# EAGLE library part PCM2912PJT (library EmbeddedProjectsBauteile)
TEXAS INSTRUMENTS PCM2912PJT - AUDIO CODEC, USB INTERFACE 32TQFP
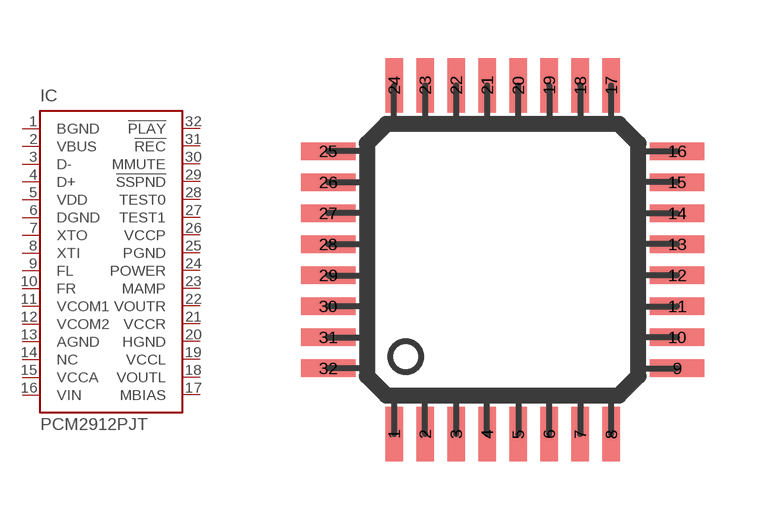
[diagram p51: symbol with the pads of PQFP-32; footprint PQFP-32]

Designator prefix IC

## PCM2912PJT  [PQFP-32]
1  BGND  pwr
2  VBUS  pwr
3  D-
4  D+
5  VDD  pwr
6  DGND  pwr
7  XTO  out
8  XTI  in
9  FL  in
10  FR  in
11  VCOM1  pwr
12  VCOM2  pwr
13  AGND  pwr
14  NC  nc
15  VCCA  pwr
16  VIN  in
17  MBIAS  out
18  VOUTL  out
19  VCCL  pwr
20  HGND  pwr
21  VCCR  pwr
22  VOUTR  out
23  MAMP  in
24  POWER  in
25  PGND  pwr
26  VCCP  pwr
27  TEST1  in
28  TEST0  in
29  !SSPND  out
30  MMUTE  in
31  !REC  out
32  !PLAY  out

## Footprint PQFP-32 (pad centres in mm)
smd 0.45 x 1.4: 1 -2.888,-4.334; 2 -2.088,-4.334; 3 -1.288,-4.334; 4 -0.488,-4.334; 5 0.312,-4.334; 6 1.112,-4.334; 7 1.912,-4.334; 8 2.712,-4.334; 17 2.712,4.666; 18 1.912,4.666; 19 1.112,4.666; 20 0.312,4.666; 21 -0.488,4.666; 22 -1.288,4.666; 23 -2.088,4.666; 24 -2.888,4.666
smd 1.4 x 0.45: 9 4.412,-2.634; 10 4.412,-1.834; 11 4.412,-1.034; 12 4.412,-0.234; 13 4.412,0.566; 14 4.412,1.366; 15 4.412,2.166; 16 4.412,2.966; 25 -4.588,2.966; 26 -4.588,2.166; 27 -4.588,1.366; 28 -4.588,0.566; 29 -4.588,-0.234; 30 -4.588,-1.034; 31 -4.588,-1.834; 32 -4.588,-2.634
